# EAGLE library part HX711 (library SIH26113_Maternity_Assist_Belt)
Avia Semiconductor HX711 24-bit ADC for bridge sensors, SOP-16L. Pin map from the HX711 English datasheet Table 1.
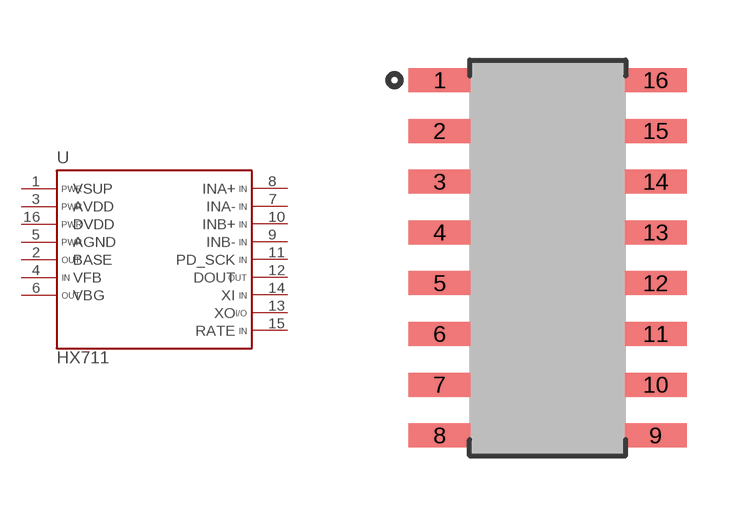
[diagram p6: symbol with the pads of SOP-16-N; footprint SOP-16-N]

Designator prefix U

## HX711  [SOP-16-N]
1  VSUP  pwr
2  BASE  out
3  AVDD  pwr
4  VFB  in
5  AGND  pwr
6  VBG  out
7  INA-  in
8  INA+  in
9  INB-  in
10  INB+  in
11  PD_SCK  in
12  DOUT  out
13  XO
14  XI  in
15  RATE  in
16  DVDD  pwr

## Footprint SOP-16-N (pad centres in mm)
SOP-16L narrow. Body 9.90 x 3.90 mm, lead span 6.00 mm, 1.27 mm pitch (HX711 datasheet Package Dimensions). Lands 1.55 x 0.60 mm at 5.40 mm span (IPC-7351B SOIC127P600X175-16N Nominal).
smd 1.55 x 0.6: 1 -2.7,4.445; 2 -2.7,3.175; 3 -2.7,1.905; 4 -2.7,0.635; 5 -2.7,-0.635; 6 -2.7,-1.905; 7 -2.7,-3.175; 8 -2.7,-4.445; 9 2.7,-4.445; 10 2.7,-3.175; 11 2.7,-1.905; 12 2.7,-0.635; 13 2.7,0.635; 14 2.7,1.905; 15 2.7,3.175; 16 2.7,4.445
